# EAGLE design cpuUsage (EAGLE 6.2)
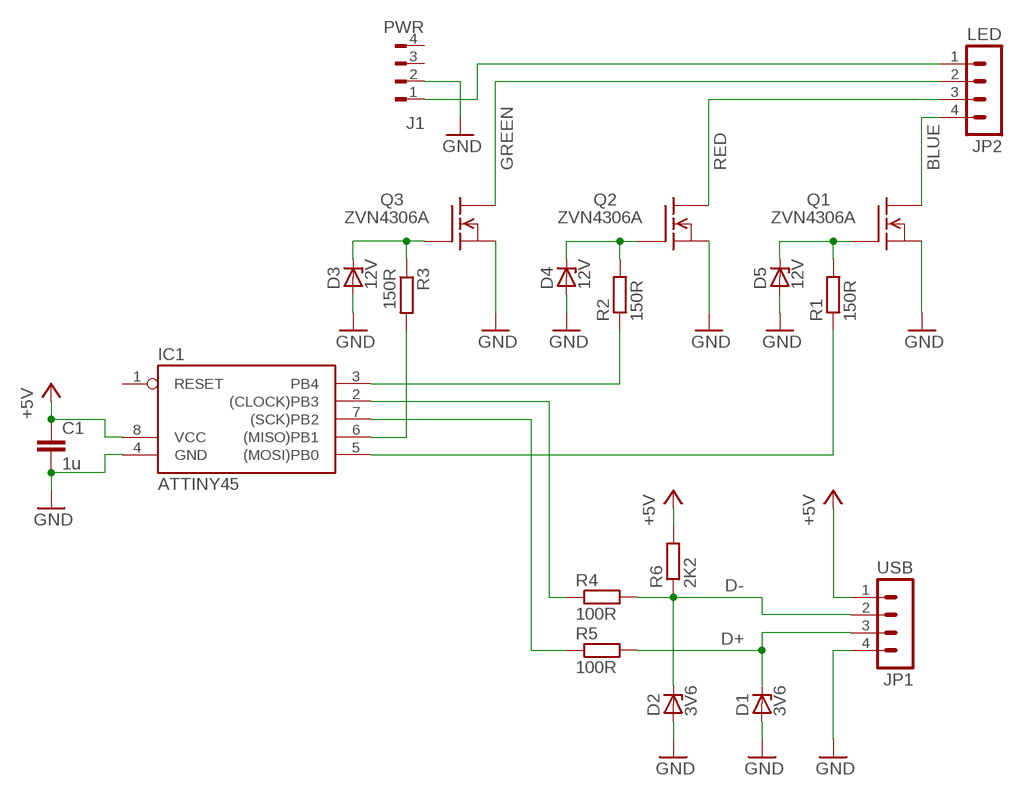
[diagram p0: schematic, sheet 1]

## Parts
C1  1u  C2.5/2  [C2.5-2]
D1  3V6  ZENER-DIODEZD-5  [ZDIO-5]
D2  3V6  ZENER-DIODEZD-5  [ZDIO-5]
D3  12V  ZENER-DIODEZD-2.5  [ZDIO-2.5]
D4  12V  ZENER-DIODEZD-2.5  [ZDIO-2.5]
D5  12V  ZENER-DIODEZD-2.5  [ZDIO-2.5]
IC1  ATTINY45  TINY22P  [DIL08]
J1  PWR  FLOP-4W827001  [827001]
JP1  USB  MA04-1  [MA04-1]
JP2  LED  MA04-1  [MA04-1]
Q1  ZVN4306A  BSS101  [TO92]
Q2  ZVN4306A  BSS101  [TO92]
Q3  ZVN4306A  BSS101  [TO92]
R1  150R  R-EU_0207/7  [0207/7]
R2  150R  R-EU_0207/7  [0207/7]
R3  150R  R-EU_0207/2V  [0207/2V]
R4  100R  R-EU_0207/7  [0207/7]
R5  100R  R-EU_0207/7  [0207/7]
R6  2K2  R-EU_0207/2V  [0207/2V]

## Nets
+5V: C1.1 IC1.8(VCC) JP1.1 R6.2
BLUE: JP2.4 Q1.3(D)
D+: D1.C JP1.3 R5.2
D-: D2.C JP1.2 R4.2 R6.1
GND: C1.2 D1.A D2.A D3.A D4.A D5.A IC1.4(GND) J1.2 JP1.4 Q1.1(S) Q2.1(S) Q3.1(S)
GREEN: JP2.2 Q3.3(D)
N$1: D3.C Q3.2(G) R3.1
N$2: D4.C Q2.2(G) R2.2
N$3: D5.C Q1.2(G) R1.2
N$7: IC1.2((CLOCK)PB3) R4.1
N$8: J1.1 JP2.1
N$9: IC1.3(PB4) R2.1
N$10: IC1.5((MOSI)PB0) R1.1
N$11: IC1.6((MISO)PB1) R3.2
N$12: IC1.7((SCK)PB2) R5.1
RED: JP2.3 Q2.3(D)
Unconnected: IC1.1(RESET) J1.3 J1.4

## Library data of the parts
C1 = capacitor-wima:C: CAPACITOR
D1-D5 = diode:ZENER-DIODE: Z-Diode
IC1 = atmel:TINY22: MICROCONTROLLER 1K ROM 128 bytes RAM 128 bytes EEPROM; OC_FARNELL: unknown; OC_NEWARK: unknown
J1 = con-amp:FLOP-4W: MATE N-LOCK Floppy / HDD conector Distributor: Bürklin 71F972
JP1 JP2 = con-lstb:MA04-1: PIN HEADER; OC_FARNELL: unknown; OC_NEWARK: unknown
Q1-Q3 = transistor-fet:BSS101: N-Channel Enhancement MOSFET 200V; 0,16A; 11Ohm
R1-R6 = resistor:R-EU_: RESISTOR, European symbol

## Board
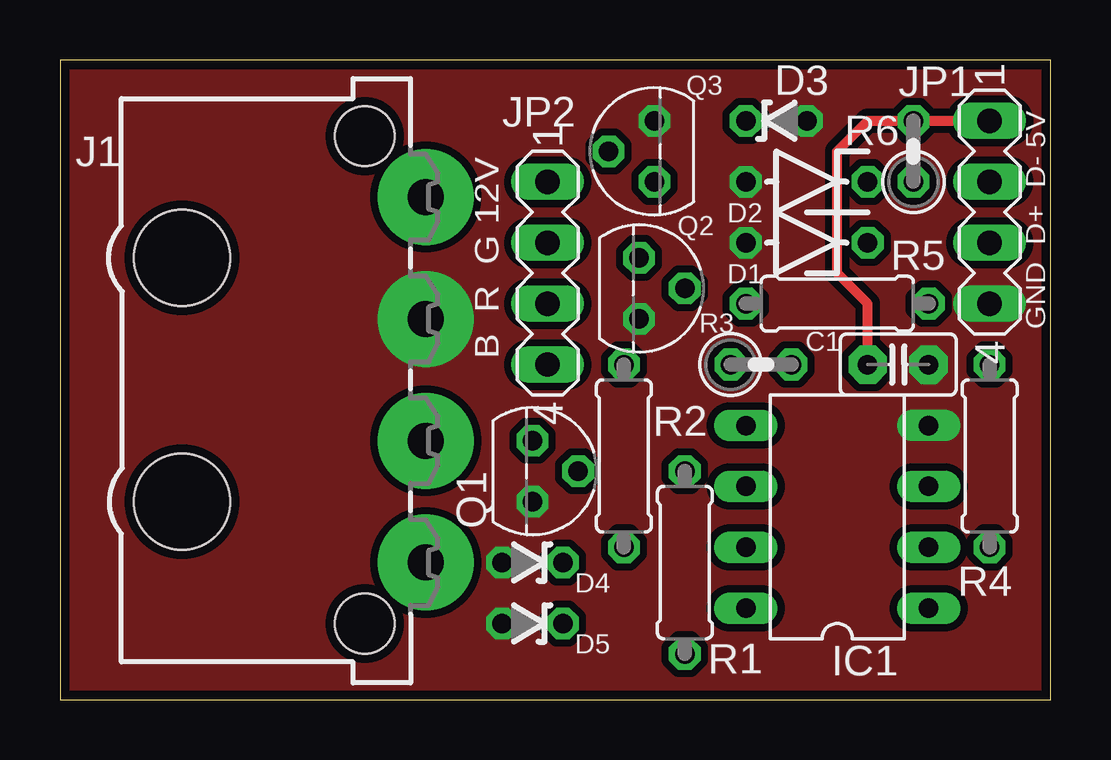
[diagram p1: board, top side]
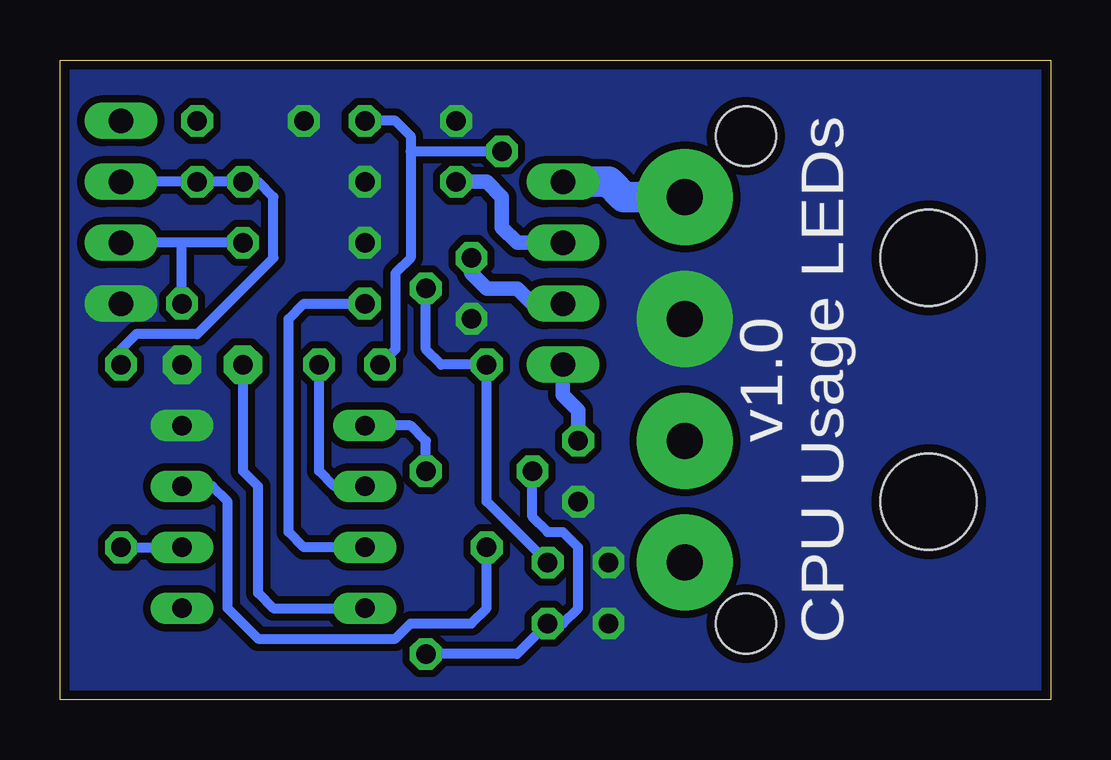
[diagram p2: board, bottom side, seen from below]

Size 41.27 x 26.67 mm. Coordinates in mm from the lower left corner, seen from the top.
Outline: 0,0 41.27,0 41.27,26.67 0,26.67 0,0
Copper layers (1*16): Top 0.0356mm / dielectric 1.5011mm / Bottom 0.0356mm
Design rules: minimum track width 6mil, minimum drill 13mil, track to track 6mil, track to pad 6mil, pad to pad 6mil, via to via 6mil, smd to smd 6mil, copper to edge 15mil, drill to drill 6mil, minimum pad ring 10mil, minimum via ring 7mil, stop-mask expansion 4mil, vias tented up to drill 0mil, thermal gap 10mil

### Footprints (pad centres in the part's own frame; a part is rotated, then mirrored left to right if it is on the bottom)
C2.5-2 = drill 0.813 pad 1.6 octagon: 1 -1.27,0; 2 1.27,0
ZDIO-5 = drill 0.813 octagon: A 2.54,0; C -2.54,0
ZDIO-2.5 = drill 0.813 octagon: A 1.27,0; C -1.27,0
DIL08 = drill 0.813 long: 1 -3.81,-3.81; 2 -1.27,-3.81; 3 1.27,-3.81; 4 3.81,-3.81; 5 3.81,3.81; 6 1.27,3.81; 7 -1.27,3.81; 8 -3.81,3.81
827001 = drill 1.5 pad 4: 1 -7.62,0; 2 -2.54,0; 3 2.54,0; 4 7.62,0 | hole 4: 5.08,-10.16; -5.08,-10.16 | hole 2.5: 10.16,-2.54; -10.16,-2.54
MA04-1 = drill 1.016 long: 1 -3.81,0; 2 -1.27,0; 3 1.27,0; 4 3.81,0
TO92 = drill 0.813 octagon: 1 1.27,0; 2 0,1.905; 3 -1.27,0
0207/7 = drill 0.813 octagon: 1 -3.81,0; 2 3.81,0
0207/2V = drill 0.813 octagon: 1 -1.27,0; 2 1.27,0

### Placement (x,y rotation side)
C1  34.92,13.97 0 top
D1  31.11,19.05 180 top
D2  31.11,21.59 180 top
D3  29.84,24.13 0 top
D4  19.68,5.71 180 top
D5  19.68,3.17 180 top
IC1  32.38,7.62 90 top
J1  15.24,13.34 270 top
JP1  38.73,20.32 270 top
JP2  20.32,17.78 270 top
Q1  19.68,9.53 270 top
Q2  24.13,17.14 270 top
Q3  24.77,22.86 90 top
R1  26.04,5.71 270 top
R2  23.5,10.16 90 top
R3  29.21,13.97 0 top
R4  38.73,10.16 90 top
R5  32.38,16.51 0 top
R6  35.56,22.86 90 top

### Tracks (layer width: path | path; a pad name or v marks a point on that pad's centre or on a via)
+5V
  Top 0.406: C1.1 33.66,16.51 32.38,17.78 32.38,22.86 33.66,24.13 R6.2 JP1.1
  Bottom 0.406: IC1.8 32.38,3.81 33.02,4.45 33.02,8.89 33.66,9.53 C1.1
BLUE
  Bottom 0.61: JP2.4 20.32,12.7 19.68,12.06 Q1.3
D+
  Bottom 0.406: R5.2 36.2,19.05 | 36.2,19.05 JP1.3 | D1.C 36.2,19.05
D-
  Bottom 0.406: JP1.2 R6.1 D2.C 33.02,21.59 32.38,20.95 32.38,18.41 35.56,15.24 38.1,15.24 38.73,14.61 R4.2
GND
  pour Bottom (isolate 0.305, no thermals): 0,26.67 41.27,26.67 41.27,0 0,0
  pour Top (isolate 0.305, no thermals): 0,26.67 41.27,26.67 41.27,0 0,0
GREEN
  Bottom 0.61: JP2.2 22.23,19.05 22.86,19.68 22.86,20.95 23.5,21.59 Q3.3
N$1
  Bottom 0.406: 26.67,22.86 Q3.2 | 26.67,22.86 26.67,23.5 27.3,24.13 D3.C | 26.67,22.86 26.67,18.41 27.3,17.78 27.3,14.61 R3.1
N$2
  Bottom 0.406: Q2.2 26.04,14.61 25.4,13.97 R2.2 23.5,8.26 D4.C
N$3
  Bottom 0.406: Q1.2 21.59,7.62 20.95,6.99 20.32,6.99 19.68,6.35 19.68,3.81 20.32,3.17 D5.C 22.23,1.91 R1.2
N$7
  Bottom 0.406: R4.1 IC1.2
N$8
  Bottom 1.27: J1.1 17.78,20.95 18.41,21.59 JP2.1
N$9
  Bottom 0.406: IC1.3 34.92,8.89 34.29,8.26 34.29,3.81 33.02,2.54 27.3,2.54 26.67,3.17 24.13,3.17 23.5,3.81 R2.1
N$10
  Bottom 0.406: IC1.5 26.67,11.43 26.04,10.79 R1.1
N$11
  Bottom 0.406: IC1.6 29.84,8.89 30.48,9.53 R3.2
N$12
  Bottom 0.406: IC1.7 31.11,6.35 31.75,6.99 31.75,15.88 31.11,16.51 R5.1
RED
  Bottom 0.61: Q2.3 24.13,17.78 23.5,17.14 22.23,17.14 21.59,16.51 JP2.3

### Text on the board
tNames: GND D+ D- 5V | B R G 12V
bNames: CPU Usage LEDs | v1.0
